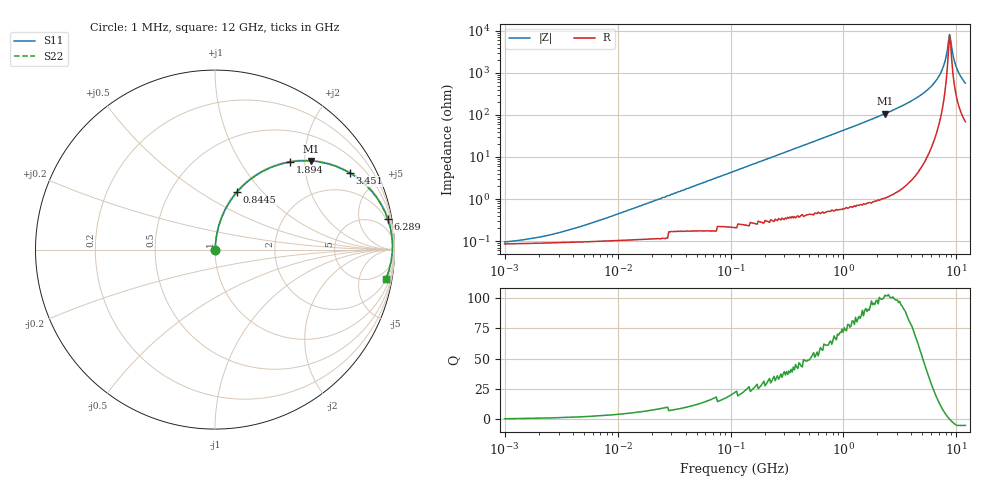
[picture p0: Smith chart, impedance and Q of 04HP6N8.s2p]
# MHz S MA R 50
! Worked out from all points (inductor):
!   408 points, 1 MHz to 12 GHz, reference 50 ohm
!   read as one part in series: L = 6.8 nH near 7.111 MHz
!   highest Q = 101 at 2.331 GHz (marker M1), where L = 7.32 nH
!   self-resonance near 8.687 GHz
!   S11 on the Smith chart (normalised r, x): 1 MHz: 1.00, +0.00; 844.5 MHz: 1.01, +0.73; 1.894 GHz: 1.02, +1.70; 3.451 GHz: 1.04, +3.50; 6.289 GHz: 1, +11; 12 GHz: 2, -11
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1  0.0008323 30.8  0.999 -0.0  0.999 -0.0  0.0008323 30.8
2.142  0.001209 49.1  0.999 -0.1  0.999 -0.1  0.001209 49.1
4.803  0.002244 65.9  0.999 -0.1  0.999 -0.1  0.002244 65.9
23.071  0.009935 81.7  0.999 -0.6  0.999 -0.6  0.009935 81.7
110.816  0.047 84.5  0.997 -2.7  0.997 -2.7  0.047 84.5
532.275  0.222 76.1  0.971 -12.8  0.971 -12.8  0.222 76.1
844.475  0.341 69.2  0.935 -19.9  0.935 -19.9  0.341 69.2
1893.985  0.644 49.3  0.758 -40.1  0.758 -40.1  0.644 49.3
2331.2  0.728 42.7  0.679 -46.7  0.679 -46.7  0.728 42.7
2556.642  0.763 39.7  0.639 -49.7  0.639 -49.7  0.763 39.7
3451.144  0.864 29.6  0.494 -59.8  0.494 -59.8  0.864 29.6
4878.67  0.945 18.1  0.311 -70.8  0.311 -70.8  0.945 18.1
6288.537  0.977 10.1  0.175 -77.6  0.175 -77.6  0.977 10.1
7057.687  0.985 6.5  0.113 -79.2  0.113 -79.2  0.985 6.5
7563.627  0.988 4.4  0.076 -78.6  0.076 -78.6  0.988 4.4
7920.912  0.989 2.9  0.052 -76.0  0.052 -76.0  0.989 2.9
8488.733  0.989 0.8  0.018 -51.5  0.018 -51.5  0.989 0.8
8686.912  0.988 0.1  0.012 -11.4  0.012 -11.4  0.988 0.1
9097.259  0.987 -1.3  0.025 58.9  0.025 58.9  0.987 -1.3
9526.989  0.985 -2.7  0.048 70.9  0.048 70.9  0.985 -2.7
10209.94  0.981 -4.8  0.084 74.7  0.084 74.7  0.981 -4.8
12000  0.966 -9.6  0.169 73.4  0.169 73.4  0.966 -9.6
